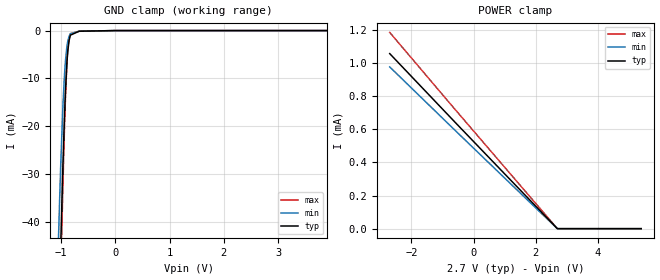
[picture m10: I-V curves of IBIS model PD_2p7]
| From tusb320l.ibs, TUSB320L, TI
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|   Model
[Model]   PD_2p7
Model_type   Input
Vinl = 0.81
Vinh = 1.89
|   typ   min   max
C_comp   0.475pF   0.451pF   0.489pF
[Voltage Range]   2.7   2.699   2.701
[Temperature Range]   27   105   -40
[Power Clamp Reference]   2.7   2.699   2.701
[GND Clamp Reference]   0   0   0
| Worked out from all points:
|   GND clamp passes 1 mA (typ) near -0.83 V on its own axis
[GND Clamp]
|   Voltage   I(typ)   I(min)   I(max)
-2.7V     -997.9mA   -935.8mA   -1.04A
-1.056V   -67.21mA   -46.46mA   -75.66mA
-1.04V    -59.5mA    -39.98mA   -67.28mA
-1.007V   -44.73mA   -28.04mA   -51.04mA
-966.6mV  -28mA      -15.7mA    -32.17mA
-942.3mV  -19.34mA   -10.11mA   -22.07mA
-918mV    -12.16mA   -6.03mA    -13.46mA
-893.7mV  -6.822mA   -3.37mA    -6.952mA
-877.5mV  -4.35mA    -2.233mA   -4.03mA
-828.9mV  -960uA     -658uA     -634.4uA
-2.7mV    -518.7nA   -477.7nA   -582.9nA
5.4V      0A         0A         0A
[POWER Clamp]
|   Voltage   I(typ)   I(min)   I(max)
-2.7V     1.056mA    976uA      1.184mA
-610.2mV  645.1uA    596.1uA    722.8uA
2.695V    1.044uA    783.3nA    1.39uA
5.4V      0A         0A         0A
